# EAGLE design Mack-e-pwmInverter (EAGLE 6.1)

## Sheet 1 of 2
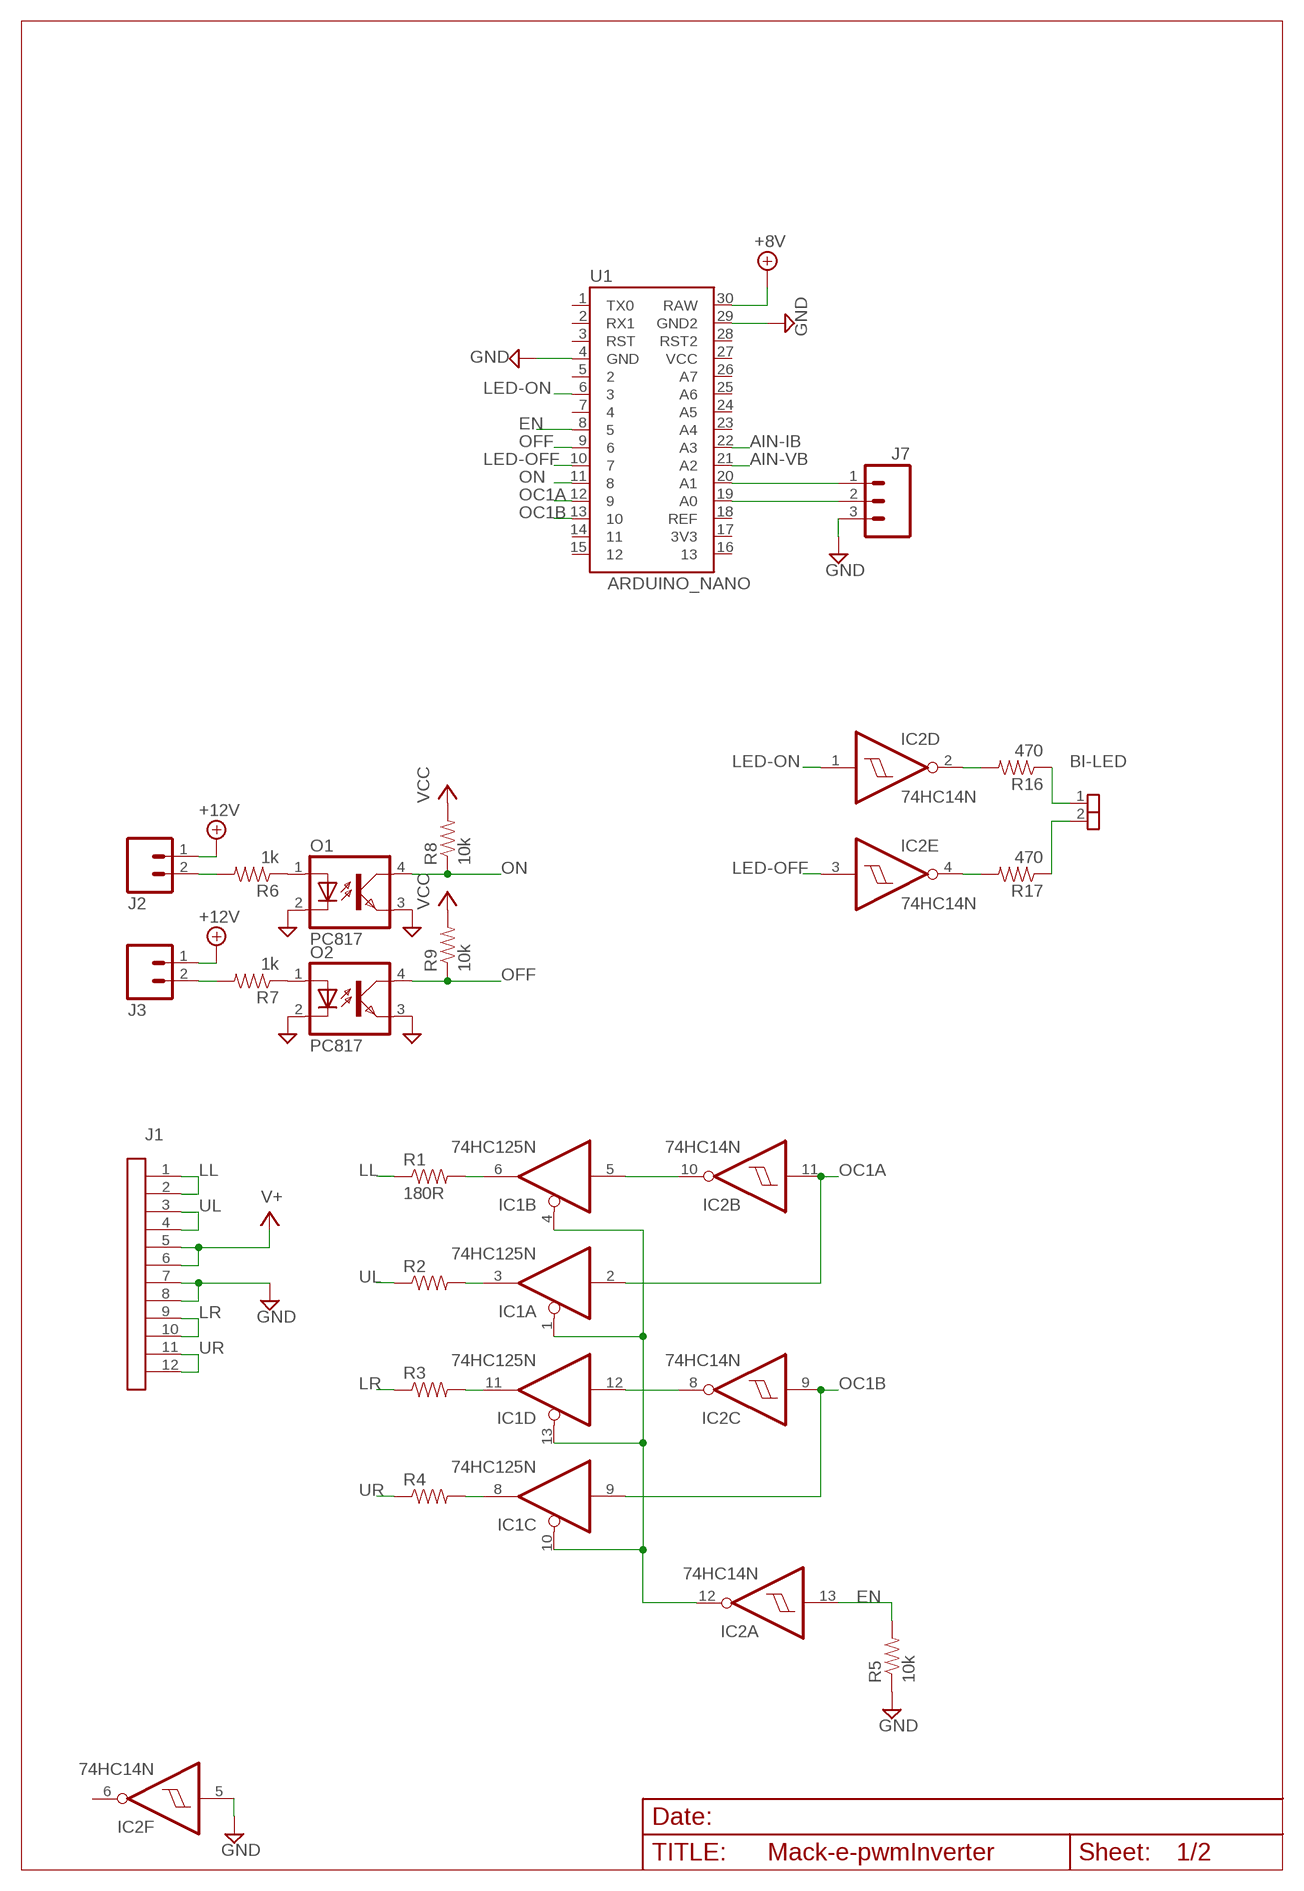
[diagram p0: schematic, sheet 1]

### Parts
BI-LED  SIL-2  [JP1]
IC1  74HC125N  [DIL14]
IC2  74HC14N  [DIL14]
J1  IDC12  [IDC12]
J2  MO2POL  [MOLEX-1X2]
J3  MO2POL  [MOLEX-1X2]
J7  MO3POL  [MOLEX-3]
O1  PC817  [DIL04]
O2  PC817  [DIL04]
R1  180R  R4  [AXIAL-0.4]
R2  R4  [AXIAL-0.4]
R3  R4  [AXIAL-0.4]
R4  R4  [AXIAL-0.4]
R5  10k  R4  [AXIAL-0.4]
R6  1k  R4  [AXIAL-0.4]
R7  1k  R4  [AXIAL-0.4]
R8  10k  R4  [AXIAL-0.4]
R9  10k  R4  [AXIAL-0.4]
R16  470  R4  [AXIAL-0.4]
R17  470  R4  [AXIAL-0.4]
U1  ARDUINO_NANO  [ARDUINO_MINI]

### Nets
+8V: U1.30(RAW) ; also sheet 2
+12V: J2.1 J3.1 ; also sheet 2
AIN-IB: U1.22(A3) ; also sheet 2
AIN-VB: U1.21(A2) ; also sheet 2
EN: IC2.13(A:I) R5.P$2 U1.8
GND: IC2.5(F:I) J1.7 J1.8 J7.3 O1.2(C) O1.3(EMIT) O2.2(C) O2.3(EMIT) R5.P$1 U1.4(GND) U1.29(GND2) ; also sheet 2
LED-OFF: IC2.3(E:I) U1.10
LED-ON: IC2.1(D:I) U1.6
LL: J1.1 J1.2 R1.P$1
LR: J1.9 J1.10 R3.P$1
N$1: O1.1(A) R6.P$1
N$2: O2.1(A) R7.P$1
N$3: J2.2 R6.P$2
N$4: J3.2 R7.P$2
N$5: IC1.6(B:O) R1.P$2
N$6: IC1.3(A:O) R2.P$2
N$7: IC1.11(D:O) R3.P$2
N$8: IC1.8(C:O) R4.P$2
N$9: IC1.5(B:I) IC2.10(B:O)
N$11: IC1.12(D:I) IC2.8(C:O)
N$13: IC1.1(A:OE) IC1.4(B:OE) IC1.10(C:OE) IC1.13(D:OE) IC2.12(A:O)
N$14: J7.1 U1.20(A1)
N$16: J7.2 U1.19(A0)
N$21: IC2.2(D:O) R16.P$2
N$22: IC2.4(E:O) R17.P$2
N$23: BI-LED.1 R16.P$1
N$24: BI-LED.2 R17.P$1
OC1A: IC1.2(A:I) IC2.11(B:I) U1.12
OC1B: IC1.9(C:I) IC2.9(C:I) U1.13
OFF: O2.4(COL) R9.P$1 U1.9
ON: O1.4(COL) R8.P$1 U1.11
UL: J1.3 J1.4 R2.P$1
UR: J1.11 J1.12 R4.P$1
V+: J1.5 J1.6 ; also sheet 2
VCC: R8.P$2 R9.P$2 ; also sheet 2
Unconnected: IC2.6(F:O) U1.1(TX0) U1.2(RX1) U1.3(RST) U1.5 U1.7 U1.14 U1.15 U1.16 U1.17(3V3) U1.18(REF) U1.23(A4) U1.24(A5) U1.25(A6) U1.26(A7) U1.27(VCC) U1.28(RST2)

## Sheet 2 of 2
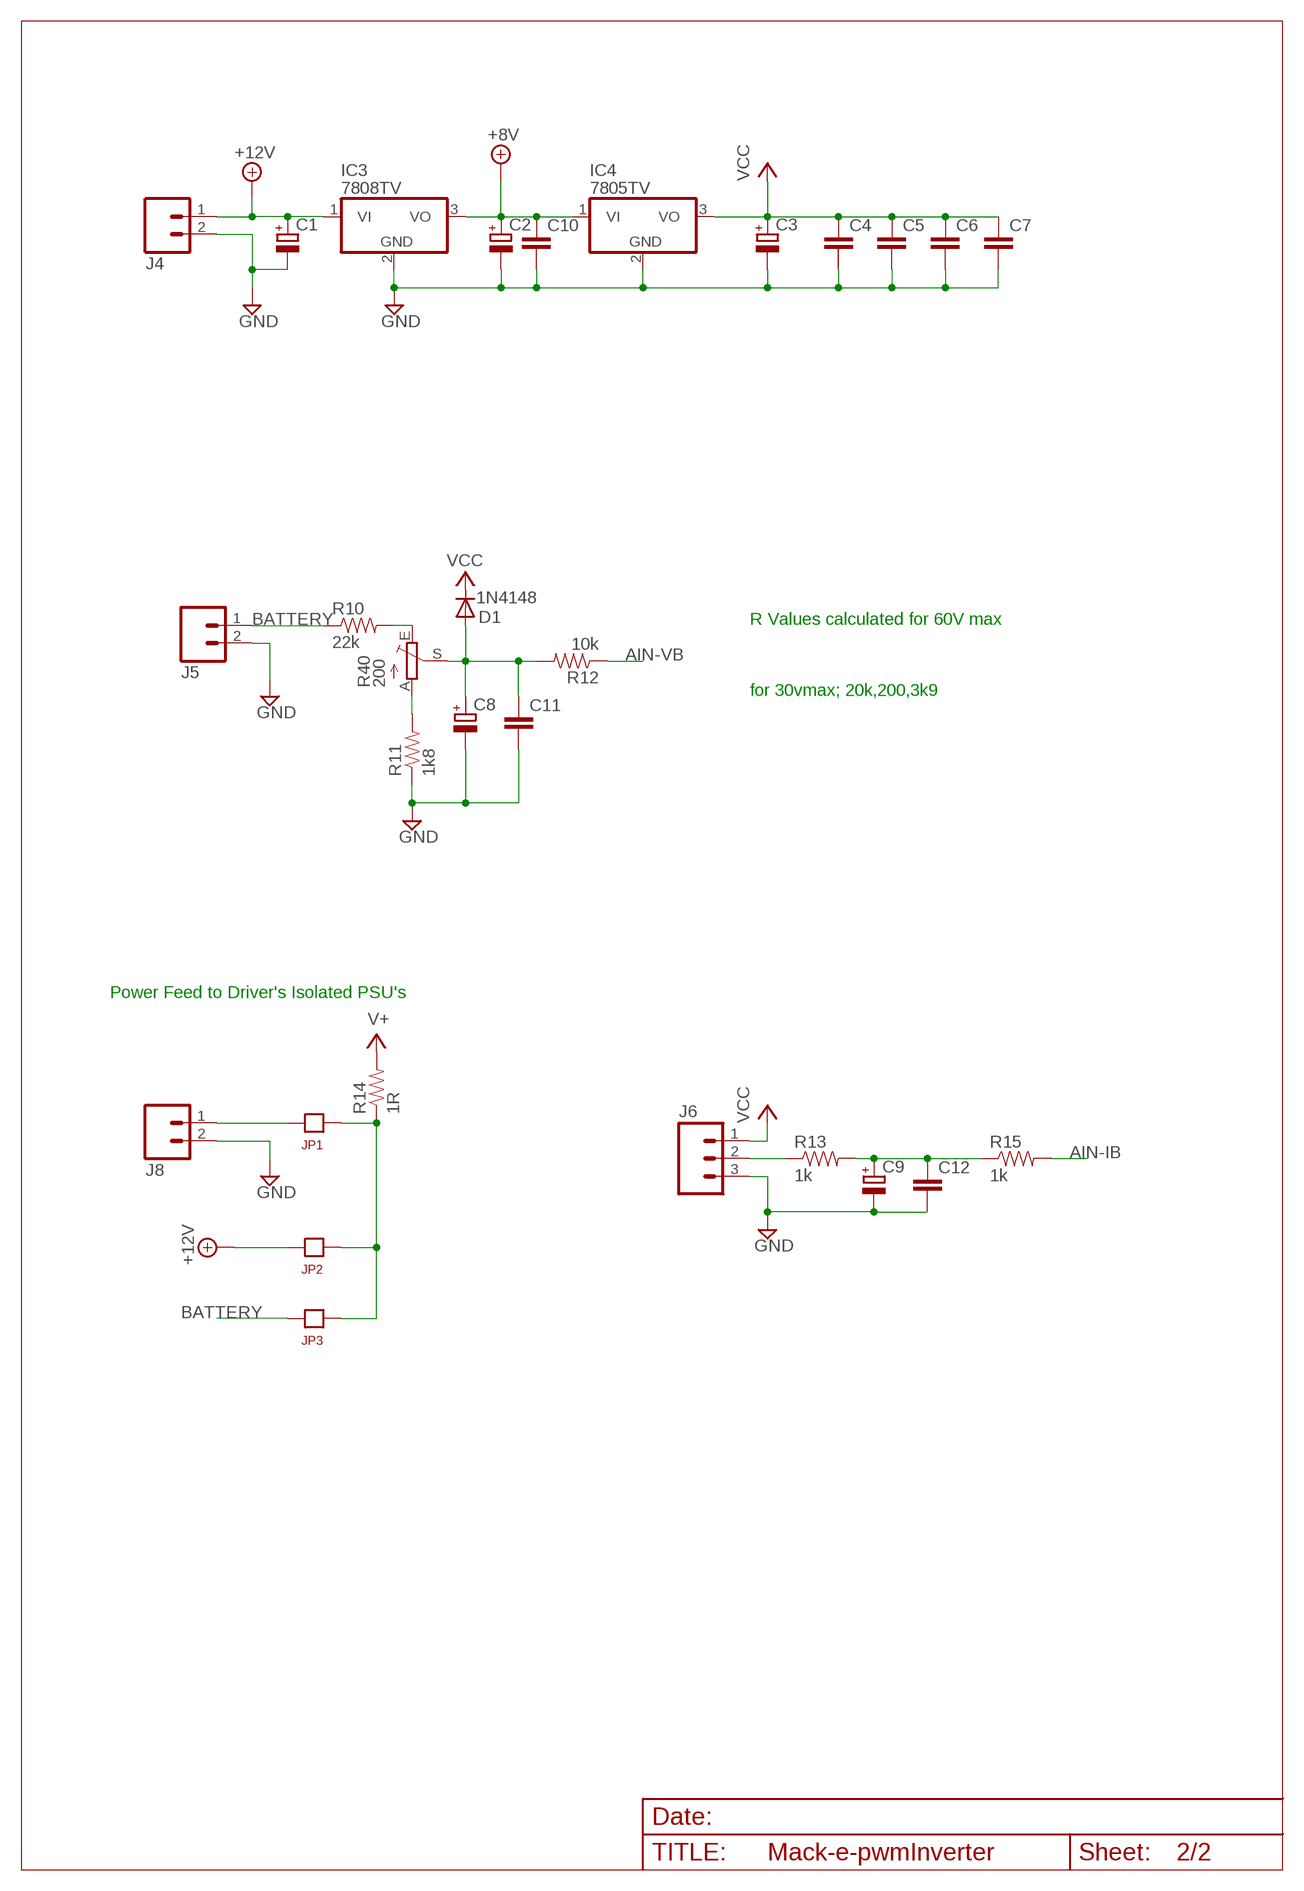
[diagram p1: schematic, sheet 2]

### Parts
C1  C-RB200100  [CPOL-RADIAL-10UF-25V]
C2  C-RB200100  [CPOL-RADIAL-10UF-25V]
C3  C-RB200100  [CPOL-RADIAL-10UF-25V]
C4  BCAP  [BCAP]
C5  BCAP  [BCAP]
C6  BCAP  [BCAP]
C7  BCAP  [BCAP]
C8  CPOL-EUE2.5-5  [E2,5-5]
C9  CPOL-EUE2.5-5  [E2,5-5]
C10  BCAP  [BCAP]
C11  BCAP  [BCAP]
C12  BCAP  [BCAP]
D1  1N4148  1N4148DO35-7  [D3]
IC3  7808TV  [TO220V]
IC4  7805TV  [TO220V]
J4  MO2POL  [MOLEX-1X2]
J5  MO2POL  [MOLEX-1X2]
J6  MO3POL  [MOLEX-3]
J8  MO2POL  [MOLEX-1X2]
JP1  JP1  [JP1]
JP2  JP1  [JP1]
JP3  JP1  [JP1]
R10  22k  R4  [AXIAL-0.4]
R11  1k8  R4  [AXIAL-0.4]
R12  10k  R4  [AXIAL-0.4]
R13  1k  R4  [AXIAL-0.4]
R14  1R  R4  [AXIAL-0.4]
R15  1k  R4  [AXIAL-0.4]
R40  200  TRIM_EU-B64Y  [B64Y]

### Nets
+8V: C2.1(+) C10.1 IC3.3(VO) IC4.1(VI) ; also sheet 1
+12V: C1.1(+) IC3.1(VI) J4.1 JP2.2 ; also sheet 1
AIN-IB: R15.P$2 ; also sheet 1
AIN-VB: R12.P$1 ; also sheet 1
BATTERY: J5.1 JP3.2 R10.P$1
GND: C1.2(-) C2.2(-) C3.2(-) C4.2 C5.2 C6.2 C7.2 C8.- C9.- C10.2 C11.2 C12.2 IC3.2(GND) IC4.2(GND) J4.2 J5.2 J6.3 J8.2 R11.P$1 ; also sheet 1
N$10: R10.P$2 R40.E
N$12: J6.2 R13.P$1
N$15: C8.+ C11.1 D1.A R12.P$2 R40.S
N$17: J8.1 JP1.2
N$18: JP1.1 JP2.1 JP3.1 R14.P$1
N$19: R11.P$2 R40.A
N$20: C9.+ C12.1 R13.P$2 R15.P$1
V+: R14.P$2 ; also sheet 1
VCC: C3.1(+) C4.1 C5.1 C6.1 C7.1 D1.C IC4.3(VO) J6.1 ; also sheet 1

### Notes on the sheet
- R Values calculated for 60V max
- for 30vmax; 20k,200,3k9
- Power Feed to Driver's Isolated PSU's

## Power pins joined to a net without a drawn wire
GND: IC1.7(P:GND) IC2.7(P:GND)
VCC: IC1.14(P:VCC) IC2.14(P:VCC)

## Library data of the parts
BI-LED = Andrew_Connectors:SIL-2
C1-C3 = Andrew:C-RB200100
C4-C7 C10-C12 = Andrew Misc:BCAP
C8 C9 = rcl:CPOL-EU: POLARIZED CAPACITOR, European symbol
D1 = Andrew Misc:1N4148: DIODE
IC1 = 74xx-eu:74*125: Quad bus BUFFER, 3-state
IC2 = 74xx-eu:74*14: Hex schmitt trigger INVERTER
IC3 IC4 = Andrew Linear:78*: Positive VOLTAGE REGULATOR Source: http://cache.national.com/ds/LM/LM78L05.pdf http://www.fairchildsemi.com/ds/LM/LM7805.pdf
J1 = Andrew_Connectors:IDC12
J2-J5 J8 = Andrew_Connectors:MO2POL
J6 J7 = Andrew_Connectors:MO3POL
JP1-JP3 = Andrew_Connectors:JP1
O1 O2 = Andrew:PC817: SHARP OPTO COUPLER; MPN: PC817X4J000F; OC_FARNELL: 9707727; OC_NEWARK: 97K7059
R1-R17 = Andrew Misc:R4
R40 = pot:TRIM_EU-: POTENTIOMETER
U1 = Andrew Misc:ARDUINO_NANO: Arduino Pro Mini footprint

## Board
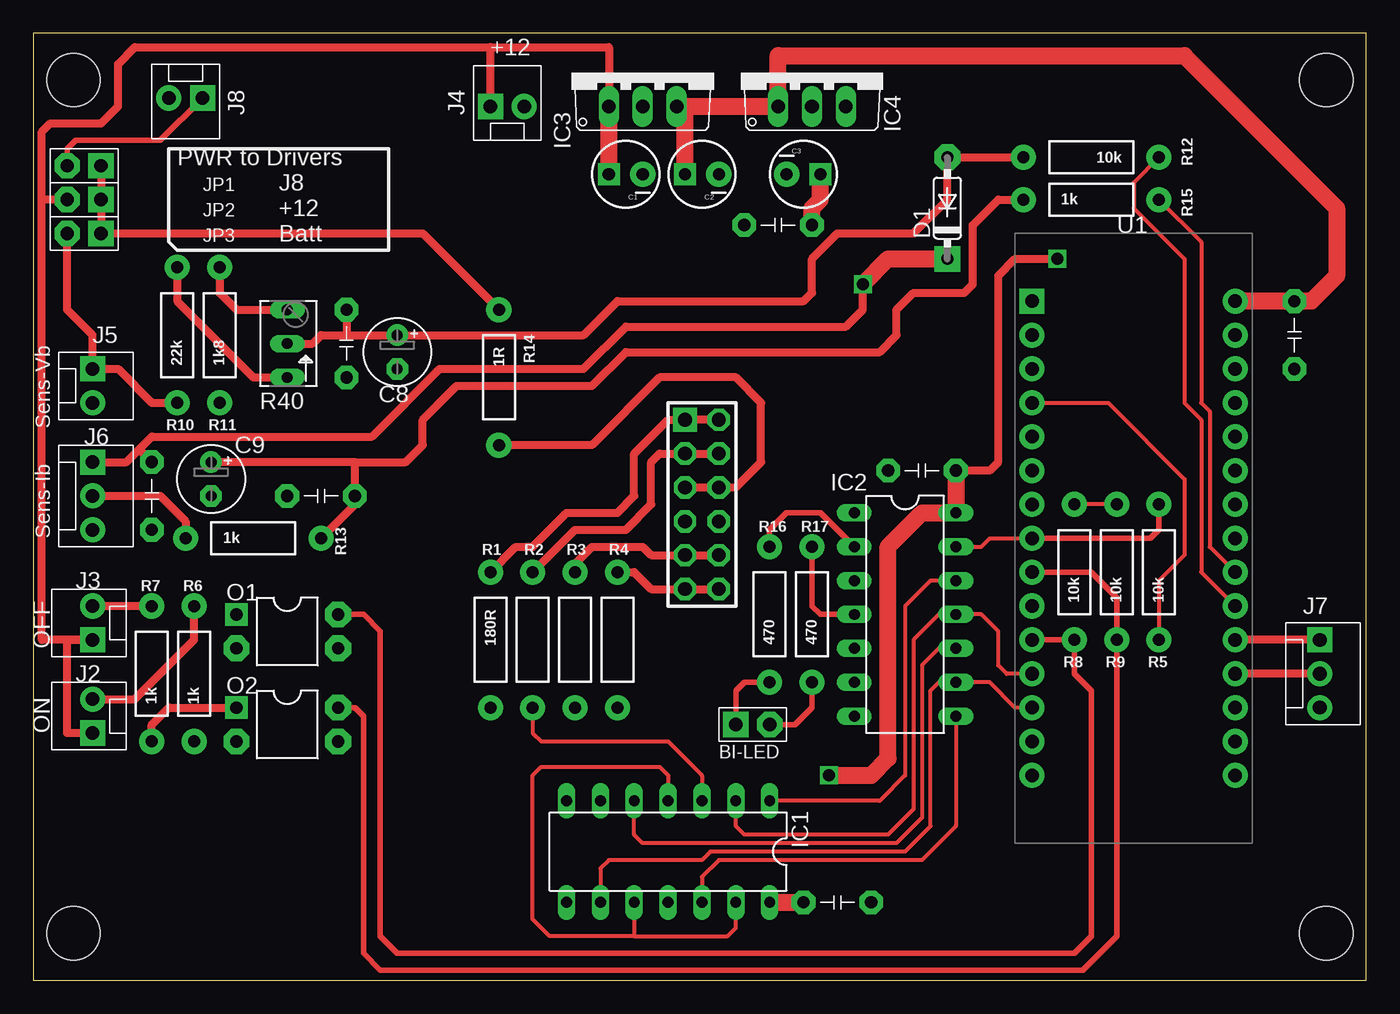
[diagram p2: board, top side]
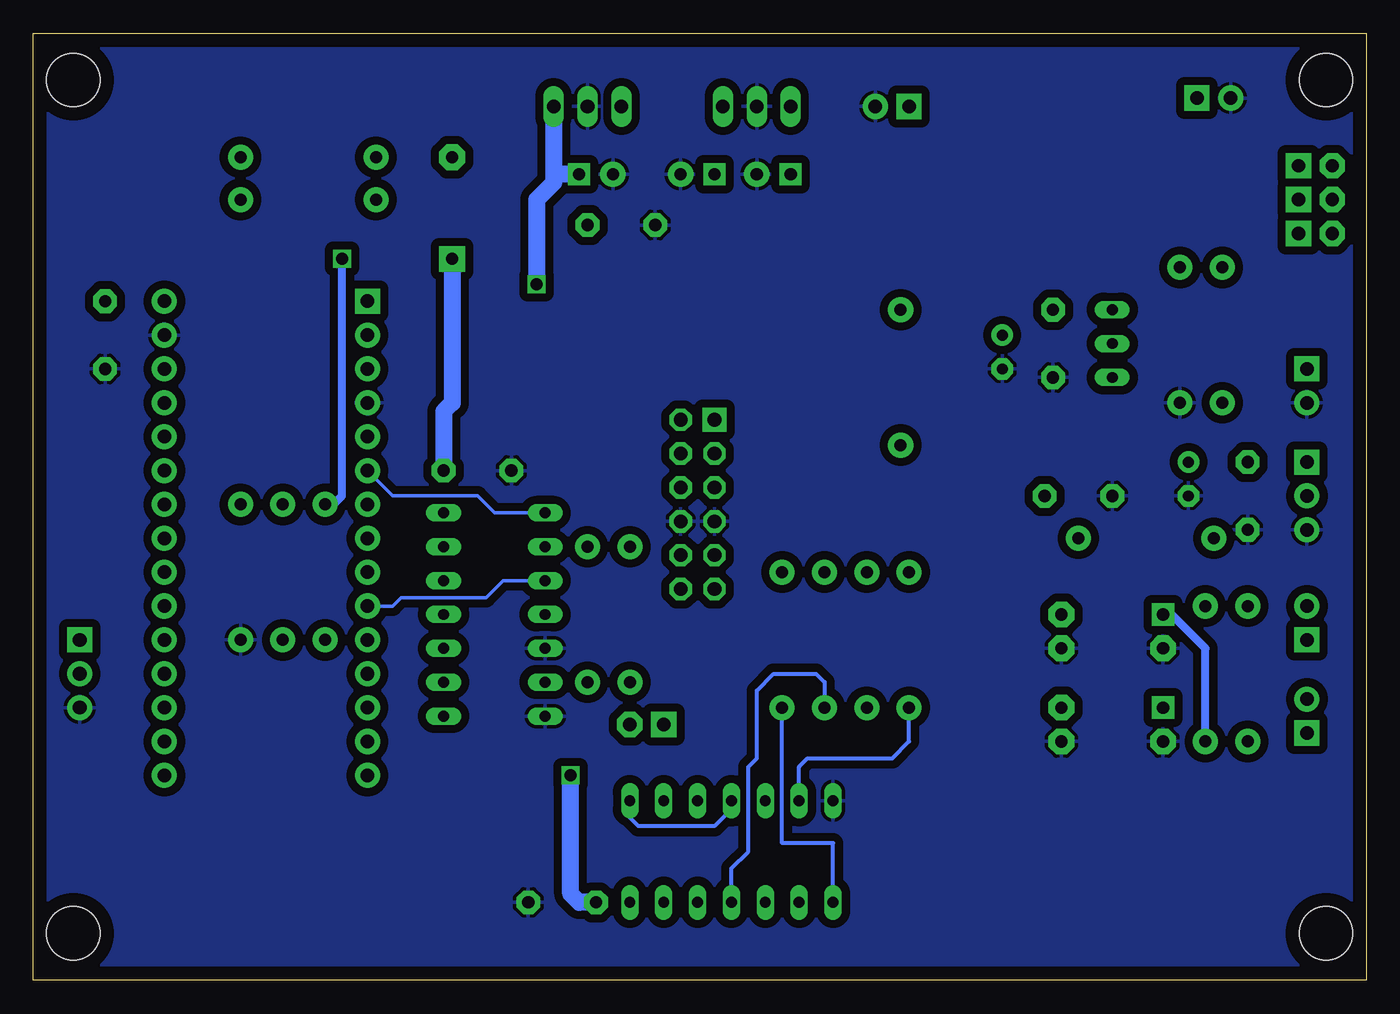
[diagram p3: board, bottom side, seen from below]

Size 100 x 71.02 mm. Coordinates in mm from the lower left corner, seen from the top.
Outline: 0,0 100,0 100,71.02 0,71.02 0,0
Copper layers (1*16): Top 0.035mm / dielectric 1.5mm / Bottom 0.035mm
Design rules: minimum track width 10mil, minimum drill 24mil, track to track 8mil, track to pad 8mil, pad to pad 8mil, via to via 8mil, smd to smd 8mil, copper to edge 40mil, drill to drill 8mil, minimum pad ring 10mil, minimum via ring 8mil, stop-mask expansion 4mil, vias tented up to drill 0mil, thermal gap 10mil
Holes 4 mm at 3,3.52 3,67.52 97,67.52 97,3.52

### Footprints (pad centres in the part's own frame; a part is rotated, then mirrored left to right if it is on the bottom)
JP1 = drill 1 pad 1.905 square: 1 -1.27,0 | drill 1 pad 1.905 octagon: 2 1.27,0
CPOL-RADIAL-10UF-25V = drill 0.914 pad 1.651 square: 1 1.27,0 | drill 0.914 pad 1.905: 2 -1.27,0
BCAP = drill 0.914 pad 1.778 octagon: 1 -2.54,0; 2 2.54,0
E2,5-5 = drill 0.813 pad 1.6: + -1.27,0 | drill 0.813 pad 1.6 octagon: - 1.27,0
D3 = drill 0.914 pad 1.93 octagon: A 3.81,0 | drill 0.914 pad 1.93 square: C -3.81,0
DIL14 = drill 0.813 long: 1 -7.62,-3.81; 2 -5.08,-3.81; 3 -2.54,-3.81; 4 0,-3.81; 5 2.54,-3.81; 6 5.08,-3.81; 7 7.62,-3.81; 8 7.62,3.81; 9 5.08,3.81; 10 2.54,3.81; 11 0,3.81; 12 -2.54,3.81; 13 -5.08,3.81; 14 -7.62,3.81
TO220V = drill 1.016 long: 1 -2.54,-2.54; 2 0,-2.54; 3 2.54,-2.54
IDC12 = drill 1.016 pad 1.778 square: 1 -1.27,6.35 | drill 1.016 pad 1.676 octagon: 2 1.27,6.35; 3 -1.27,3.81; 4 1.27,3.81; 5 -1.27,1.27; 6 1.27,1.27; 7 -1.27,-1.27; 8 1.27,-1.27; 9 -1.27,-3.81; 10 1.27,-3.81; 11 -1.27,-6.35; 12 1.27,-6.35
MOLEX-1X2 = drill 1.016 pad 1.88 square: 1 0,0 | drill 1.016 pad 1.88: 2 2.54,0
MOLEX-3 = drill 1.016 pad 1.88 square: 1 -2.54,0 | drill 1.016 pad 1.88: 2 0,0; 3 2.54,0
DIL04 = drill 0.914 pad 1.676 square: 1 -1.27,-3.81 | drill 0.914 pad 1.93 octagon: 2 1.27,-3.81; 3 1.27,3.81; 4 -1.27,3.81
AXIAL-0.4 = drill 0.9 pad 1.88: P$1 -5.08,0; P$2 5.08,0
B64Y = drill 0.813 long: A 2.54,0; E -2.54,0; S 0,0
ARDUINO_MINI = drill 1.016 pad 1.88 square: 1 -7.62,12.7 | drill 1.016 pad 1.88: 2 -7.62,10.16; 3 -7.62,7.62; 4 -7.62,5.08; 5 -7.62,2.54; 6 -7.62,0; 7 -7.62,-2.54; 8 -7.62,-5.08; 9 -7.62,-7.62; 10 -7.62,-10.16; 11 -7.62,-12.7; 12 -7.62,-15.24; 13 -7.62,-17.78; 14 -7.62,-20.32; 15 -7.62,-22.86; 16 7.62,-22.86; 17 7.62,-20.32; 18 7.62,-17.78; 19 7.62,-15.24; 20 7.62,-12.7; 21 7.62,-10.16; 22 7.62,-7.62; 23 7.62,-5.08; 24 7.62,-2.54; 25 7.62,0; 26 7.62,2.54; 27 7.62,5.08; 28 7.62,7.62; 29 7.62,10.16; 30 7.62,12.7

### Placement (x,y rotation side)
BI-LED  53.98,19.18 0 top
C1  44.45,60.45 180 top
C2  50.16,60.45 180 top
C3  57.78,60.45 0 top
C4  55.88,56.64 180 top
C5  8.89,36.32 270 top
C6  66.67,38.23 180 top
C7  60.33,5.84 0 top
C8  27.3,47.12 270 top
C9  13.34,37.59 270 top
C10  94.61,48.39 270 top
C11  23.5,47.75 270 top
C12  21.59,36.32 180 top
D1  68.58,57.91 90 top
IC1  47.62,9.65 180 top
IC2  65.41,27.43 270 top
IC3  45.72,68.07 0 top
IC4  58.42,68.07 0 top
J1  50.16,35.69 0 top
J2  4.45,18.54 90 top
J3  4.45,25.53 90 top
J4  34.29,65.53 0 top
J5  4.45,45.85 270 top
J6  4.45,36.32 270 top
J7  96.52,22.99 270 top
J8  12.7,66.17 180 top
JP1  3.81,61.09 180 top
JP2  3.81,58.55 180 top
JP3  3.81,56.01 180 top
O1  19.05,26.16 270 top
O2  19.05,19.18 270 top
R1  34.29,25.53 270 top
R2  37.47,25.53 270 top
R3  40.64,25.53 270 top
R4  43.81,25.53 270 top
R5  84.45,30.61 90 top
R6  12.06,22.99 90 top
R7  8.89,22.99 90 top
R8  78.11,30.61 90 top
R9  81.28,30.61 90 top
R10  10.79,48.39 90 top
R11  13.97,48.39 90 top
R12  79.38,61.72 180 top
R13  16.51,33.15 0 top
R14  34.92,45.21 270 top
R15  79.38,58.55 0 top
R16  55.24,27.43 90 top
R17  58.42,27.43 90 top
R40  19.05,47.75 90 top
U1  82.55,38.23 0 top

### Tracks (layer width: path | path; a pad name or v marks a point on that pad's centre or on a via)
+8V
  Top 1.27: IC3.3 48.9,65.53 | 48.9,65.53 IC4.1 55.88,69.34 86.36,69.34 97.79,57.91 97.79,52.83 95.89,50.93 95.25,50.93 C10.1 U1.30 | C2.1 48.9,65.53
+12V
  Top 0.61: J2.1 2.54,18.54 2.54,25.53 J3.1 0.64,25.53 0.64,58.55 | 0.64,58.55 0.64,63.63 1.27,64.26 5.08,64.26 6.35,65.53 6.35,68.71 7.62,69.98 34.29,69.98 | 34.29,69.98 43.18,69.98 IC3.1 | J4.1 34.29,69.98 | JP2.2 0.64,58.55
  Top 1.27: C1.1 IC3.1
AIN-IB
  Top 0.305: R15.P$2 87.63,55.37 87.63,43.31 88.27,42.67 88.27,32.51 U1.22
AIN-VB
  Top 0.305: R12.P$1 82.55,59.82 82.55,57.91 86.36,54.1 86.36,43.31 87.63,42.04 87.63,30.61 U1.21
BATTERY
  Top 0.61: JP3.2 2.54,50.29 4.45,48.39 J5.1 6.35,45.85 8.89,43.31 R10.P$1
EN
  Top 0.305: IC2.13 71.12,32.51 71.75,33.15 U1.8
  Top 0.406: U1.8 83.82,33.15 84.45,33.78 R5.P$2
GND
  Top 0.305: U1.4 80.64,43.31 86.36,37.59 86.36,31.88 84.45,29.97 R5.P$1
  pour Bottom (isolate 0.61): 0.64,70.61 99.69,70.61 99.69,0.76 0.64,0.76
LED-OFF
  Bottom 0.254: IC2.3 64.77,29.97 66.04,28.7 72.39,28.7 73.03,28.07 U1.10
LED-ON
  Bottom 0.254: IC2.1 65.41,35.05 66.67,36.32 73.03,36.32 U1.6
LL
  Top 0.61: R1.P$1 36.2,32.51 37.47,32.51 40.01,35.05 43.81,35.05 45.09,36.32 45.09,39.5 47.62,42.04 J1.1 J1.2
LR
  Top 0.61: R3.P$1 40.64,31.24 41.91,32.51 45.72,32.51 46.35,31.88 J1.9 J1.10
N$1
  Bottom 0.61: R6.P$1 12.06,24.89 14.61,27.43 O1.1
N$2
  Top 0.61: R7.P$1 8.89,19.18 10.16,20.45 O2.1
N$3
  Top 0.61: J2.2 7.62,21.08 12.06,25.53 R6.P$2
N$4
  Top 0.61: R7.P$2 J3.2
N$5
  Bottom 0.305: IC1.6 42.55,16 41.91,16.64 35.56,16.64 34.29,17.91 R1.P$2
N$6
  Top 0.305: R2.P$2 37.47,18.54 38.1,17.91 47.62,17.91 50.16,15.37 IC1.3
N$7
  Bottom 0.305: IC1.11 47.62,8.38 46.35,9.65 46.35,16 45.72,16.64 45.72,21.72 44.45,22.99 41.27,22.99 40.64,22.35 R3.P$2
N$8
  Bottom 0.305: IC1.8 40.01,10.29 43.81,10.29 R4.P$2
N$9
  Top 0.305: IC2.10 67.94,24.89 66.67,23.62 66.67,12.19 64.77,10.29 45.72,10.29 45.09,10.92 IC1.5
N$10
  Top 0.61: R10.P$2 10.79,50.93 16.51,45.21 R40.E
N$11
  Top 0.305: IC2.8 69.22,11.56 66.67,9.02 51.44,9.02 50.16,7.75 IC1.12
N$12
  Top 0.61: J6.2 9.53,36.32 11.43,34.42 R13.P$1
N$13
  Top 0.305: IC1.10 45.09,3.3 | 45.09,3.3 52.07,3.3 52.7,3.94 IC1.13 | IC2.12 67.31,29.97 65.41,28.07 65.41,15.37 63.5,13.46 IC1.1 | 45.09,3.3 38.73,3.3 37.47,4.57 37.47,15.37 38.1,16 46.99,16 47.62,15.37 IC1.4
  Bottom 0.305: IC1.4 47.62,12.83 48.9,11.56 54.61,11.56 55.24,12.19 IC1.1
N$14
  Top 0.61: J7.1 U1.20
N$15
  Top 0.61: R40.S 20.95,47.75 21.59,48.39 23.5,48.39 | 23.5,48.39 C8.+ 41.27,48.39 43.81,50.93 57.78,50.93 58.42,51.56 58.42,54.1 60.33,56.01 66.04,56.01 68.58,58.55 D1.A R12.P$2 | C11.1 23.5,48.39
N$16
  Top 0.61: J7.2 U1.19
N$17
  Top 0.406: J8.1 9.53,62.99 3.17,62.99 2.54,62.36 JP1.2
N$18
  Top 0.61: JP1.1 JP2.1 JP3.1 29.21,56.01 R14.P$1
N$19
  Top 0.61: R11.P$2 13.97,51.56 15.24,50.29 R40.A
N$20
  Top 0.61: R13.P$2 24.13,35.69 C12.1 24.13,38.86 | 24.13,38.86 C9.+ | 24.13,38.86 27.94,38.86 29.21,40.13 29.21,42.04 31.75,44.58 41.91,44.58 44.45,47.12 63.5,47.12 64.77,48.39 64.77,50.29 66.04,51.56 69.85,51.56 70.48,52.2 70.48,56.64 72.39,58.55 R15.P$1
N$21
  Top 0.406: R16.P$2 55.24,33.78 56.52,35.05 59.05,35.05 IC2.2
N$22
  Top 0.406: R17.P$2 58.42,28.07 59.05,27.43 IC2.4
N$23
  Top 0.406: R16.P$1 53.34,22.35 52.7,21.72 BI-LED.1
N$24
  Top 0.406: BI-LED.2 57.15,19.18 58.42,20.45 R17.P$1
OC1A
  Top 0.305: U1.12 73.03,22.99 72.39,23.62 72.39,26.16 71.12,27.43 IC2.11 67.94,27.43 66.04,25.53 66.04,12.83 64.14,10.92 53.34,10.92 52.7,11.56 IC1.2
OC1B
  Top 0.305: U1.13 73.66,20.45 71.75,22.35 IC2.9 67.94,22.35 67.31,21.72 67.31,11.56 65.41,9.65 50.8,9.65 50.16,9.02 43.18,9.02 42.55,8.38 IC1.9
OFF
  Top 0.406: O2.4 24.13,20.45 24.77,19.81 24.77,2.03 26.04,0.76 78.74,0.76 81.28,3.3 R9.P$1 81.28,28.7 79.38,30.61 U1.9
ON
  Top 0.406: U1.11 R8.P$1 78.11,22.99 79.38,21.72 79.38,3.3 78.11,2.03 27.3,2.03 26.04,3.3 26.04,26.16 24.77,27.43 O1.4
UL
  Top 0.61: R2.P$1 40.64,33.78 44.45,33.78 46.35,35.69 46.35,38.86 46.99,39.5 J1.3 J1.4
UR
  Top 0.61: R4.P$1 45.09,30.61 46.35,29.34 J1.11 J1.12
V+
  Top 0.61: J1.6 J1.5 52.7,36.96 54.61,38.86 54.61,43.31 52.7,45.21 46.99,45.21 41.91,40.13 R14.P$2
VCC  (via drill 0.9)
  Top 0.305: R9.P$2 R8.P$2
  Top 0.61: J6.1 6.99,38.86 7.94,39.81 | v62.23,52.2 62.23,50.29 60.96,49.02 44.45,49.02 41.27,45.85 30.48,45.85 25.4,40.77 8.89,40.77 7.94,39.81 | C5.1 7.94,39.81 | C6.1 71.75,38.23 72.39,38.86 72.39,52.83 73.66,54.1 v76.83,54.1
  Top 1.27: IC1.14 C7.1 | v59.69,15.37 62.87,15.37 64.14,16.64 64.14,32.51 66.67,35.05 IC2.14 C6.1 | v62.23,52.2 64.14,54.1 D1.C | C4.1 58.42,57.91 59.05,58.55 C3.1
  Bottom 0.61: R8.P$2 77.47,35.69 76.83,36.32 v76.83,54.1
  Bottom 1.27: C7.1 59.05,5.84 59.69,6.48 v59.69,15.37 | D1.C 68.58,43.31 69.22,42.67 C6.1 | IC4.3 60.96,60.45 | 60.96,60.45 60.96,59.82 62.23,58.55 v62.23,52.2 | C3.1 60.96,60.45

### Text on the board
tPlace: +12 | PWR to Drivers | J8 | +12 | Batt | Sens-Vb | Sens-Ib | OFF | ON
